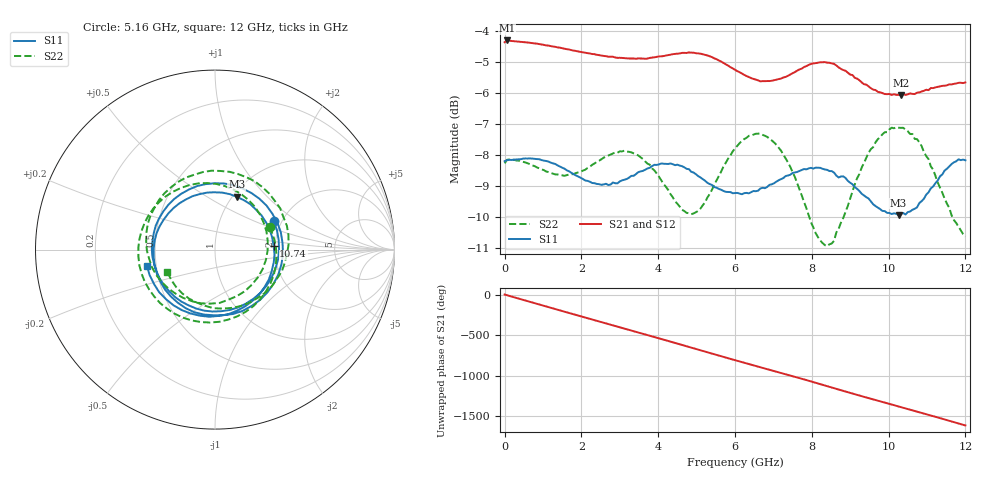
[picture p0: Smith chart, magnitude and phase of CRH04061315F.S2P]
!Agilent Technologies,E5071C,MY46109174,A.10.05
!Date: Wed Jun 26 07:23:55 2013
!Data & Calibration Information:
!Freq	S11:SOLT2(ON)	S21:SOLT2(ON)	S12:SOLT2(ON)	S22:SOLT2(ON)
!PortZ  Port1:50+j0  Port2:50+j0
!Above PortZ is port z conversion or system Z0 setting when saving the data.
!When reading, reference impedance value at option line is always used.
# Hz S dB R 50
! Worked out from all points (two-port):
!   201 points, 300 kHz to 12 GHz, reference 50 ohm
!   highest |S21| = -4.31 dB at 60.3 MHz (marker M1); lowest = -6.1 dB at 10.32 GHz (marker M2)
!   |S21| within 3 dB of the highest: start of sweep to end of sweep
!   lowest |S11| = -9.9 dB at 10.26 GHz (marker M3), VSWR 1.93, Z = 52.4 + j34.3 ohm
!   |S11| at or under -10 dB: nowhere
!   |S22| runs from -11.0 to -7.1 dB; largest |S21 - S12| = 0.0034
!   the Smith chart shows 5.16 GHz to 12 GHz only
!   S11 on the Smith chart (normalised r, x): 5.16 GHz: 1.81, +0.67; 10.74 GHz: 1.97, +0.08; 12 GHz: 0.44, -0.10
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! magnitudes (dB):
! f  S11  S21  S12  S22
! 300 kHz  -8.2  -4.4  -4.4  -8.3
! 60.3 MHz  -8.2  -4.3  -4.3  -8.2
! 900.3 MHz  -8.1  -4.4  -4.4  -8.4
! 2.04 GHz  -8.8  -4.7  -4.7  -8.5
! 3.12 GHz  -8.8  -4.9  -4.9  -7.9
! 4.02 GHz  -8.3  -4.8  -4.8  -8.7
! 4.74 GHz  -8.5  -4.7  -4.7  -9.9
! 5.16 GHz  -8.8  -4.8  -4.7  -9.6
! 6 GHz  -9.2  -5.3  -5.2  -7.8
! 6.54 GHz  -9.2  -5.6  -5.6  -7.3
! 7.02 GHz  -8.9  -5.6  -5.6  -7.6
! 7.44 GHz  -8.6  -5.4  -5.4  -8.4
! 8.04 GHz  -8.4  -5.1  -5.0  -10.3
! 8.34 GHz  -8.5  -5.0  -5.0  -10.9
! 8.58 GHz  -8.6  -5.1  -5.1  -10.8
! 9.48 GHz  -9.4  -5.8  -5.7  -7.9
! 10.02 GHz  -9.9  -6.0  -6.1  -7.2
! 10.26 GHz  -9.9  -6.1  -6.1  -7.1
! 10.32 GHz  -9.9  -6.1  -6.1  -7.1
! 10.74 GHz  -9.7  -6.0  -6.0  -7.5
! 11.46 GHz  -8.5  -5.8  -5.8  -9.4
! 12 GHz  -8.2  -5.7  -5.7  -10.6
